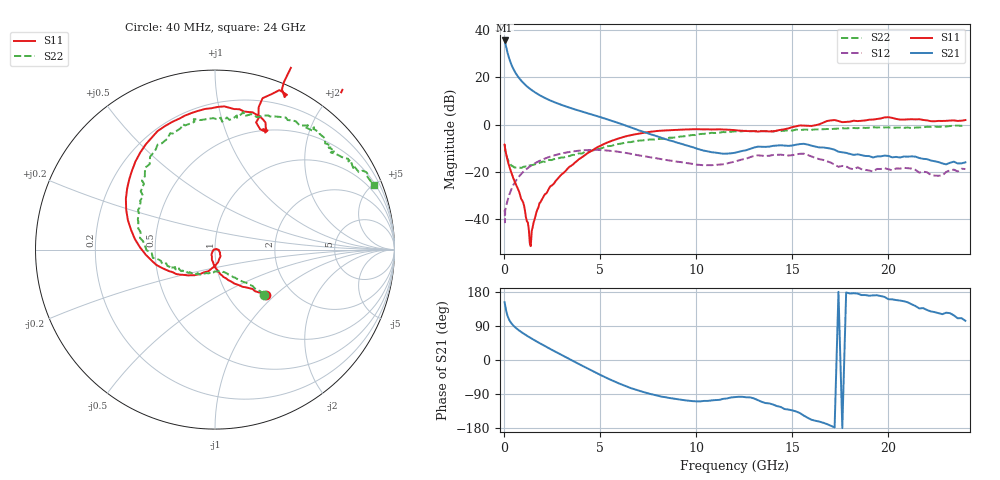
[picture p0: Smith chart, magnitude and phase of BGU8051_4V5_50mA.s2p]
! BGU8051_4V5_50mA
! Date/time Tue Jun 16 11:08:37 2015
! VAR V_out= 4.5000
! VAR I_out= 50.0100
! VAR V_in= 5.5100
! VAR I_in= 0.6818
# MHz S MA R 50
!  Freq-MHz  S11-mag  S11-arg  S21-mag  S21-arg  S12-mag  S12-arg  S22-mag  S22-arg
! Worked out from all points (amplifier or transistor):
!   187 points, 40 MHz to 24 GHz, reference 50 ohm
!   highest |S21| = 35.6 dB at 40 MHz (marker M1)
!   |S21| within 3 dB of that: start of sweep to 126.9 MHz
!   unconditionally stable (mu >= 1): 55.97 MHz to 63.58 MHz; 405.1 MHz to 13.36 GHz; 13.42 GHz to 14.03 GHz
!   at 750 MHz: K = 1.02, MAG = 20.5 dB, |S12| = -22.4 dB
!   at 5.4 GHz: K = 1.19, MAG = 3.9 dB, |S12| = -11.0 dB
!   at 24 GHz: K = -0.84, MSG = 1.4 dB, |S12| = -18.8 dB
!   lowest NFmin = 0.37 dB at 400 MHz
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40  0.3772 -41.6  60.47 152.6  0.01442 35.8  0.3722 -42.5
60  0.3211 -46.1  56.27 146.7  0.008515 32.7  0.3102 -44.3
80  0.2899 -48.0  51.55 140.8  0.0158 36.6  0.2772 -45.0
120  0.2374 -56.3  43.98 130.2  0.01872 42.9  0.2336 -49.5
160  0.2004 -63.0  37.47 121.9  0.02183 50.0  0.2052 -52.9
200  0.17 -69.2  32.29 115.4  0.02578 53.7  0.184 -56.6
260  0.1401 -77.7  26.52 107.9  0.03051 57.3  0.1621 -60.4
320  0.1149 -83.1  22.32 102.3  0.03619 59.9  0.1475 -63.6
400  0.09294 -90.8  18.32 96.4  0.04358 61.0  0.1362 -67.6
500  0.07229 -97.8  14.95 90.6  0.053 61.7  0.1287 -73.3
700  0.04662 -111.5  10.88 81.5  0.0713 60.7  0.1219 -81.1
900  0.02672 -129.3  8.55 74.0  0.08951 57.9  0.1209 -90.2
1400  0.002656 38.0  5.548 58.0  0.1334 48.8  0.1378 -107.8
1500  0.006727 23.9  5.189 54.9  0.1418 46.7  0.1394 -109.9
2500  0.05147 -56.0  3.127 26.8  0.2153 25.1  0.1775 -132.6
4100  0.2078 -136.3  1.866 -15.8  0.2847 -11.0  0.247 -156.1
5400  0.419 178.1  1.281 -48.7  0.2818 -39.5  0.3493 -172.4
8200  0.7433 111.8  0.524 -96.8  0.1852 -76.1  0.4978 147.1
12200  0.7451 67.7  0.2636 -97.0  0.1737 -75.6  0.7113 103.5
16200  0.968 67.3  0.3427 -160.3  0.1965 -149.0  0.79 70.4
20200  1.383 34.2  0.2021 160.0  0.1072 -157.6  0.8524 43.9
24000  1.247 21.4  0.1587 103.5  0.1142 -176.9  0.9536 22.1
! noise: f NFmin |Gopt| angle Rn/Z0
400  0.3688  0.04353  68.99  0.0482
550  0.3748  0.04186  97.92  0.0485
950  0.4035  0.06829  145.5  0.0489
1250  0.4372  0.09412  160  0.049
1600  0.4898  0.1221  170.4  0.0493
1900  0.5463  0.1437  177.3  0.05
2250  0.6254  0.1667  184.3  0.0517
2600  0.7188  0.1881  190.7  0.0548
3300  0.9483  0.2301  202.5  0.0666
4000  1.235  0.2757  212.5  0.0889
